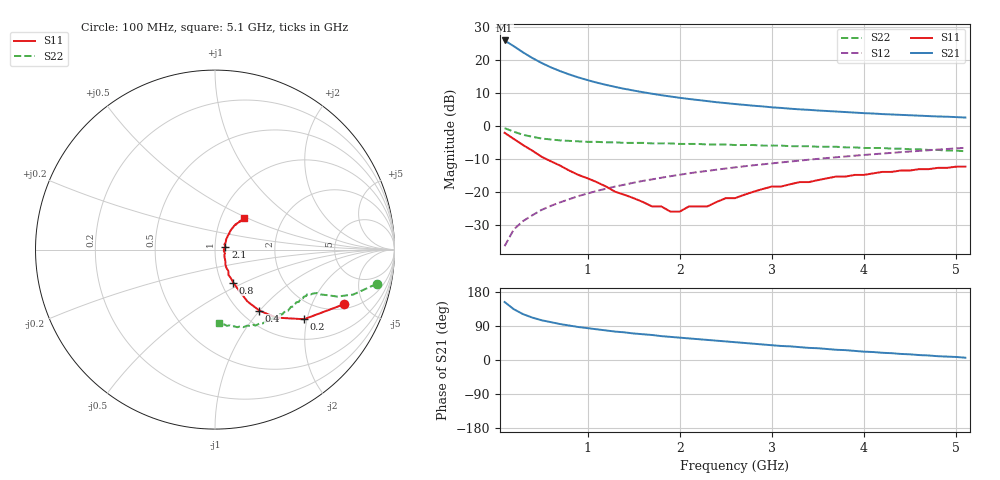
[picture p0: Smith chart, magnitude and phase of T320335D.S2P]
!AT-32033
!S PARAMETERS at Vce=5 V  Ic=7.5mA.  LAST UPDATED 01-05-95
# ghz s ma r 50
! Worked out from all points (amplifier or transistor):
!   51 points, 100 MHz to 5.1 GHz, reference 50 ohm
!   highest |S21| = 25.8 dB at 100 MHz (marker M1)
!   |S21| within 3 dB of that: start of sweep to 267.2 MHz
!   unconditionally stable (mu >= 1): 1.166 GHz to 2.448 GHz
!   at 900 MHz: K = 0.97, MSG = 18.0 dB, |S12| = -21.3 dB
!   at 2.6 GHz: K = 1.00, MSG = 9.6 dB, |S12| = -12.6 dB
!   at 5.1 GHz: K = 0.93, MSG = 4.6 dB, |S12| = -6.7 dB
!   S11 on the Smith chart (normalised r, x): 100 MHz: 2.27, -3.54; 200 MHz: 1.49, -1.92; 400 MHz: 1.21, -1.00; 800 MHz: 1.14, -0.44; 2.1 GHz: 1.12, +0.03; 5.1 GHz: 1.29, +0.48
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0.1  0.78 -23.0  19.55 153.0  0.015 78.0  0.92 -12.0
0.2  0.63 -38.0  15.99 134.0  0.027 73.0  0.81 -18.0
0.3  0.51 -48.0  12.9 121.0  0.036 71.0  0.73 -21.0
0.4  0.42 -54.0  10.62 112.0  0.044 70.0  0.68 -22.0
0.5  0.34 -58.0  8.94 105.0  0.053 70.0  0.64 -23.0
0.6  0.29 -59.0  7.68 100.0  0.061 70.0  0.62 -23.0
0.7  0.25 -60.0  6.73 95.0  0.069 70.0  0.6 -24.0
0.8  0.21 -61.0  5.99 91.0  0.077 70.0  0.59 -25.0
0.9  0.18 -61.0  5.39 87.0  0.086 70.0  0.58 -25.0
1  0.16 -62.0  4.91 84.0  0.094 70.0  0.57 -26.0
1.1  0.14 -58.0  4.49 81.0  0.103 69.0  0.57 -27.0
1.3  0.1 -55.0  3.87 75.0  0.12 68.0  0.56 -29.0
1.5  0.08 -45.0  3.41 70.0  0.137 67.0  0.55 -31.0
1.8  0.06 -21.0  2.9 63.0  0.163 65.0  0.54 -35.0
1.9  0.05 -10.0  2.77 61.0  0.172 64.0  0.54 -36.0
2.1  0.06 13.0  2.54 57.0  0.19 63.0  0.53 -38.0
2.3  0.06 29.0  2.36 53.0  0.207 61.0  0.52 -41.0
2.6  0.08 41.0  2.13 47.0  0.234 58.0  0.51 -45.0
3.1  0.12 49.0  1.86 37.0  0.278 53.0  0.5 -53.0
3.5  0.15 51.0  1.7 31.0  0.315 50.0  0.48 -59.0
4.3  0.2 49.0  1.48 18.0  0.388 42.0  0.45 -72.0
5.1  0.24 47.0  1.33 6.0  0.463 33.0  0.41 -87.0
